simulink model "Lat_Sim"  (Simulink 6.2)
settings: Solver=ode45  StartTime=0.0  StopTime=80  RelTol=1e-3
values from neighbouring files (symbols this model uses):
  r2d = 180/pi    (= 57.2957795131)    [run_lat.m]    (also in Pl.m)
undefined symbols (not defined in the file or in its folder): An, Bn, Cn, Dn, Kg

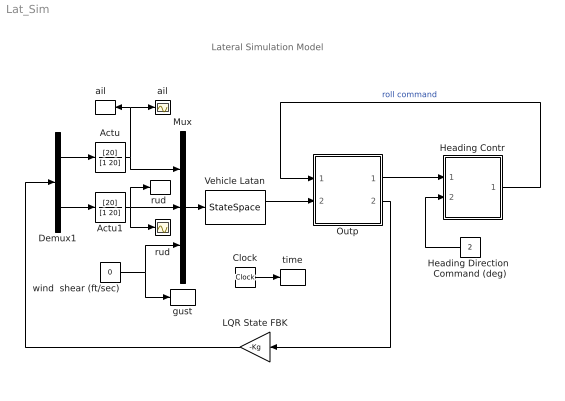
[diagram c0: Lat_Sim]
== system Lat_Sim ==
  note: Lateral Simulation Model
  Actu : TransferFcn  Numerator=[20]  Denominator=[1 20]
  Actu1 : TransferFcn  Numerator=[20]  Denominator=[1 20]
  Clock : Clock
  Demux1 : Demux  Outputs=2
  Heading Contr : Subsystem
  Heading Direction  Command (deg) : Constant  Orientation=left  Value=2
  LQR State FBK : Gain  Orientation=left  Gain=-Kg  Multiplication=Matrix(K*u) (u vector)
  Mux : Mux  Inputs=3
  Outp : Subsystem
  Vehicle Latan : StateSpace  A=An  B=Bn  C=Cn  D=Dn
  ail : Scope
  "ail   " : ToWorkspace  VariableName=ail  SampleTime=-1  SaveFormat=Array
  gust : ToWorkspace  VariableName=Gust  SampleTime=-1  SaveFormat=Array
  rud : Scope
  "rud " : ToWorkspace  VariableName=rud  SampleTime=-1  SaveFormat=Array
  time : ToWorkspace  VariableName=time  SampleTime=-1  SaveFormat=Array
  wind  shear (ft/sec) : Constant  Value=0
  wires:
  Vehicle Latan/1 -> Outp/2(out)
  Mux/1 -> Vehicle Latan/1
  Demux1/2 -> Actu1/1
  Demux1/1 -> Actu/1
  wind  shear (ft/sec)/1 -> Mux/3, gust/1
  Outp/1(Vcr) -> Heading Contr/1(Vcr)
  Actu1/1 -> Mux/2, rud/1, "rud "/1
  Actu/1 -> Mux/1, ail/1, "ail   "/1
  LQR State FBK/1 -> Demux1/1
  Outp/2(x) -> LQR State FBK/1
  Heading Direction  Command (deg)/1 -> Heading Contr/2(chi-cmd)
  Heading Contr/1(phi-cmd) -> Outp/1(phi-cmd)  "roll command"
  Clock/1 -> time/1

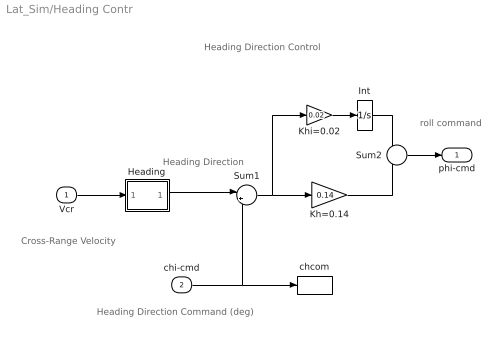
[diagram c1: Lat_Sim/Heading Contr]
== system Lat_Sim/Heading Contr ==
  note: Heading Direction Command (deg)
  note: roll command
  note: Heading Direction
  note: Heading Direction Control
  note: Cross-Range Velocity
  Vcr : Inport  Port=1  LatchInput=off
  chi-cmd : Inport  Port=2  LatchInput=off
  Heading : Subsystem
  Int : Integrator
  Kh=0.14 : Gain  Gain=0.14
  Khi=0.02 : Gain  Gain=0.02
  Sum1 : Sum  Inputs=|+-
  Sum2 : Sum  Inputs=--
  chcom : ToWorkspace  VariableName=chcom  SampleTime=-1  SaveFormat=Array
  phi-cmd : Outport
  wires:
  chi-cmd/1 -> Sum1/2, chcom/1
  Vcr/1 -> Heading/1(Vcr)
  Sum1/1 -> Khi=0.02/1, Kh=0.14/1
  Sum2/1 -> phi-cmd/1
  Int/1 -> Sum2/1
  Kh=0.14/1 -> Sum2/2
  Khi=0.02/1 -> Int/1
  Heading/1("chi ") -> Sum1/1

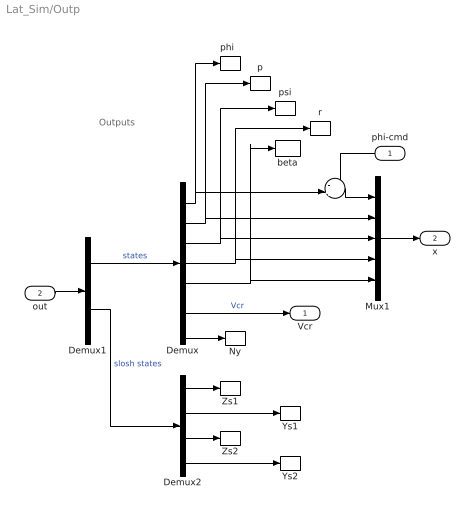
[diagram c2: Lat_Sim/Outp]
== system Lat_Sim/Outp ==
  note: Outputs
  phi-cmd : Inport  Orientation=left  Port=1  LatchInput=off
  out : Inport  Port=2  LatchInput=off
  "    " : Sum  Inputs=-+|  OutScaling=2^-10
  Demux : Demux  Outputs=7
  Demux1 : Demux  Outputs=[7, 4]
  Demux2 : Demux
  Mux1 : Mux  Inputs=5
  Ny : ToWorkspace  VariableName=Ny  SampleTime=-1  SaveFormat=Array
  Ys1 : ToWorkspace  VariableName=LYs  SampleTime=-1  SaveFormat=Array
  Ys2 : ToWorkspace  VariableName=RYs  SampleTime=-1  SaveFormat=Array
  Zs1 : ToWorkspace  VariableName=LZs  SampleTime=-1  SaveFormat=Array
  Zs2 : ToWorkspace  VariableName=RZs  SampleTime=-1  SaveFormat=Array
  beta : ToWorkspace  VariableName=beta  SampleTime=-1  SaveFormat=Array
  p : ToWorkspace  VariableName=p  SampleTime=-1  SaveFormat=Array
  "phi  " : ToWorkspace  VariableName=phi  SampleTime=-1  SaveFormat=Array
  psi : ToWorkspace  VariableName=psi  SampleTime=-1  SaveFormat=Array
  r : ToWorkspace  VariableName=r  SampleTime=-1  SaveFormat=Array
  Vcr : Outport
  x : Outport  Port=2
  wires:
  Demux/7 -> Ny/1
  Demux/5 -> Mux1/5, beta/1
  Demux/4 -> Mux1/4, r/1
  Demux/3 -> Mux1/3, psi/1
  Demux/2 -> Mux1/2, p/1
  Demux/1 -> "    "/2, "phi  "/1
  Demux/6 -> Vcr/1  "Vcr"
  Mux1/1 -> x/1
  "    "/1 -> Mux1/1
  phi-cmd/1 -> "    "/1
  Demux1/1 -> Demux/1  "states"
  out/1 -> Demux1/1
  Demux1/2 -> Demux2/1  "slosh states"
  Demux2/1 -> Zs1/1
  Demux2/3 -> Zs2/1
  Demux2/2 -> Ys1/1
  Demux2/4 -> Ys2/1

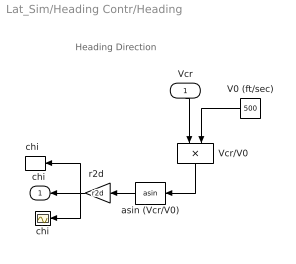
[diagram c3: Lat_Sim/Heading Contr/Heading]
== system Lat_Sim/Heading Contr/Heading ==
  note: Heading Direction
  Vcr : Inport  Orientation=down  Port=1  LatchInput=off
  V0 (ft/sec) : Constant  Orientation=left  Value=500
  Vcr/V0 : Product  Orientation=down  Inputs=*/
  asin (Vcr/V0) : Trigonometry  Orientation=left  Operator=asin
  chi : Scope
  "chi  " : ToWorkspace  VariableName=chi  SampleTime=-1  SaveFormat=Array
  "r2d " : Gain  Orientation=left  Gain=r2d
  "chi " : Outport  Orientation=left
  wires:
  Vcr/1 -> Vcr/V0/1
  V0 (ft/sec)/1 -> Vcr/V0/2
  asin (Vcr/V0)/1 -> "r2d "/1
  Vcr/V0/1 -> asin (Vcr/V0)/1
  "r2d "/1 -> "chi  "/1, chi/1, "chi "/1
